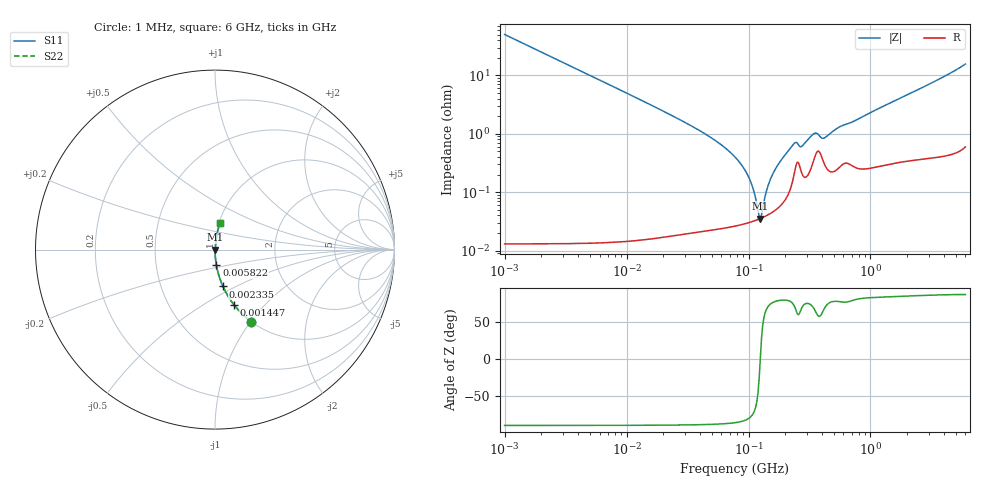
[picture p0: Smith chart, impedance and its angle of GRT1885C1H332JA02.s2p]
!Murata Part Number: GRT1885C1H332JA02
!These Parameters are Measured in Series Mode Connection
!Data Generated on Jun 19, 2026
!  o--ll--o
!Port1  Port2
!  o------o
!Operation Temp=25[degC], DC Bias Voltage=0[V]
!Freq. Start=1000[kHz] Stop=6[GHz] 401[Steps]
# Hz S RI R 50
!Freq.(Hz) S11(Real) S11(Imag) S21(Real) S21(Imag) S12(Real) S12(Imag) S22(Real) S22(Imag)
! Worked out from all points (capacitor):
!   401 points, 1 MHz to 6 GHz, reference 50 ohm
!   read as one part in series: C = 3.17 nF near 1.044 MHz
!   lowest |Z| = 35.4 mohm at 125 MHz (marker M1)
!   series resonance near 124.8 MHz, so ESL is about 510 pH
!   S11 on the Smith chart (normalised r, x): 1 MHz: 1.00, -1.00; 1.447 MHz: 1.00, -0.69; 2.335 MHz: 1.00, -0.43; 5.822 MHz: 1.00, -0.17; 6 GHz: 1.01, +0.31
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1000000  0.201 -0.4007  0.799 0.4007  0.799 0.4007  0.201 -0.4007
1447343  0.1073 -0.3093  0.8927 0.3093  0.8927 0.3093  0.1073 -0.3093
2335446  0.0442 -0.2052  0.9558 0.2052  0.9558 0.2052  0.0442 -0.2052
4293785  0.0136 -0.1151  0.9864 0.1151  0.9864 0.1151  0.0136 -0.1151
5822046  0.00746 -0.0853  0.9925 0.0853  0.9925 0.0853  0.00746 -0.0853
1.843659e7  0.000871 -0.0266  0.9991 0.0266  0.9991 0.0266  0.000871 -0.0266
4.697123e7  0.000303 -0.00915  0.9997 0.00915  0.9997 0.00915  0.000303 -0.00915
7.745967e7  0.000278 -0.00399  0.9997 0.00399  0.9997 0.00399  0.000278 -0.00399
1.005588e8  0.000304 -0.00177  0.9997 0.00177  0.9997 0.00177  0.000304 -0.00177
1.096987e8  0.00032 -0.00105  0.9997 0.00105  0.9997 0.00105  0.00032 -0.00105
1.196694e8  0.000341 -0.000343  0.9997 0.000343  0.9997 0.000343  0.000341 -0.000343
1.249896e8  0.000354 1.31e-05  0.9996 -1.31e-05  0.9996 -1.31e-05  0.000354 1.31e-05
1.305463e8  0.000368 0.000371  0.9996 -0.000371  0.9996 -0.000371  0.000368 0.000371
1.487431e8  0.000425 0.00147  0.9996 -0.00147  0.9996 -0.00147  0.000425 0.00147
1.770109e8  0.000559 0.00304  0.9994 -0.00304  0.9994 -0.00304  0.000559 0.00304
2.348496e8  0.00192 0.00642  0.9981 -0.00642  0.9981 -0.00642  0.00192 0.00642
2.734687e8  0.00213 0.00571  0.9979 -0.00571  0.9979 -0.00571  0.00213 0.00571
3.325952e8  0.00299 0.00901  0.997 -0.00901  0.997 -0.00901  0.00299 0.00901
4.224887e8  0.00298 0.00803  0.997 -0.00803  0.997 -0.00803  0.00298 0.00803
5.60538e8  0.00286 0.0128  0.9971 -0.0128  0.9971 -0.0128  0.00286 0.0128
1.428092e9  0.00408 0.0328  0.9959 -0.0328  0.9959 -0.0328  0.00408 0.0328
6e9  0.0293 0.1507  0.9707 -0.1507  0.9707 -0.1507  0.0293 0.1507
